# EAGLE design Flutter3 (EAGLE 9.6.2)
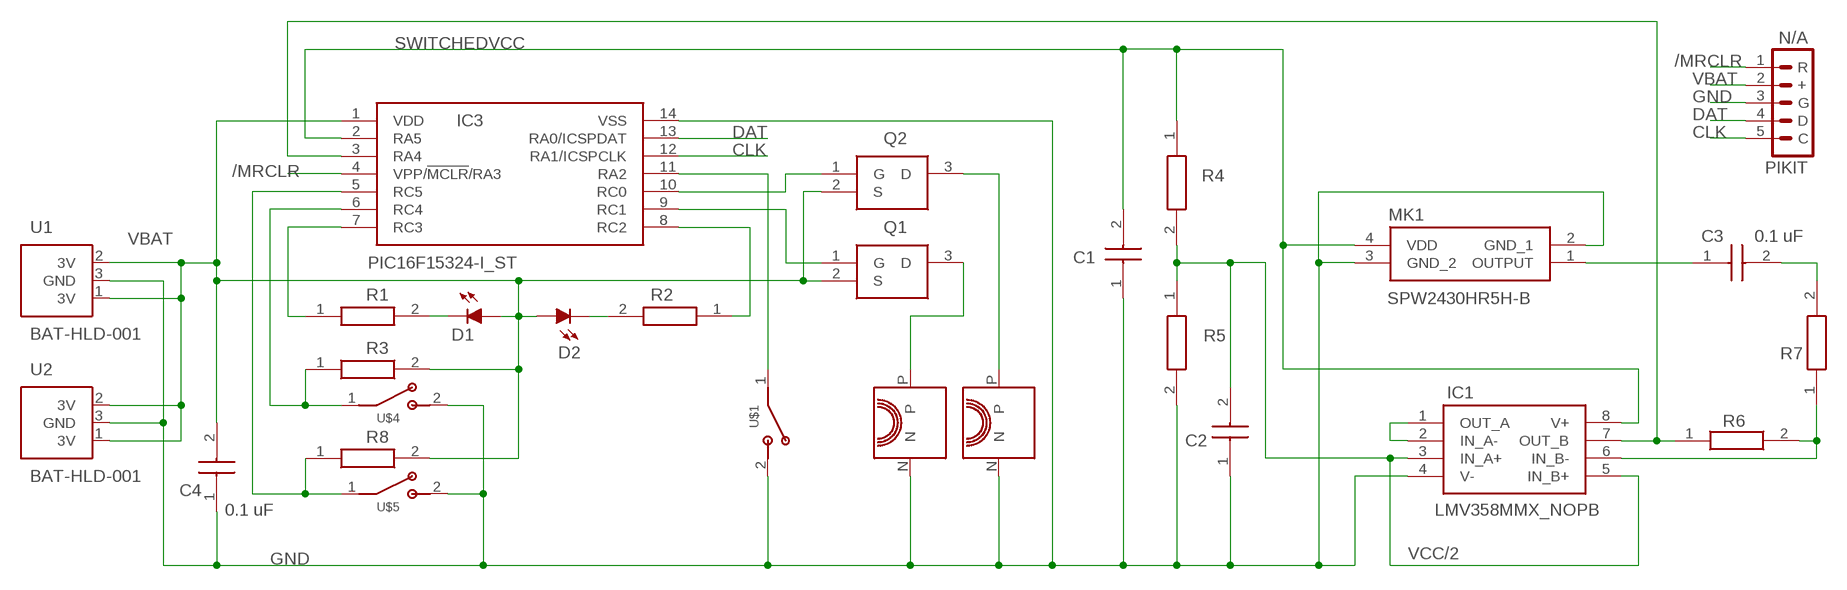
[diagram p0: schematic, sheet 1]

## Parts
C1  10 uF  C0805C106K8PACTU  [CAPC2013X140N]
C2  1.0 uF  CC0603KRX7R7BB104  [CAPC1608X90N]
C3  0.1 uF  CC0603KRX7R7BB104  [CAPC1608X90N]
C4  0.1 uF  CC0603KRX7R7BB104  [CAPC1608X90N]
D1  LEDCHIPLED_0805  [CHIPLED_0805]
D2  LEDCHIPLED_0805  [CHIPLED_0805]
IC1  LMV358MMX_NOPB  [SOP65P490X110-8N]
IC3  PIC16F15324-I_ST  [SOP65P640X120-14N]
MK1  SPW2430HR5H-B  [SPW2430HR5HB]
PIKIT  N/A  PICKIT  [MA05-1]
Q1  NTR4171PT1G  [SOT96P237X111-3N]
Q2  NTR4171PT1G  [SOT96P237X111-3N]
R1  220  CRCW0603240RFKEB  [RESC1608X50N]
R2  220  CRCW0603240RFKEB  [RESC1608X50N]
R3  220  CRCW0603240RFKEB  [RESC1608X50N]
R4  10 K  CRCW0603240RFKEB  [RESC1608X50N]
R5  10 K  CRCW0603240RFKEB  [RESC1608X50N]
R6  100 K  CRCW0603240RFKEB  [RESC1608X50N]
R7  1K  CRCW0603240RFKEB  [RESC1608X50N]
R8  220  CRCW0603240RFKEB  [RESC1608X50N]
U1  BAT-HLD-001  [BATHLD001]
U2  BAT-HLD-001  [BATHLD001]
U$1  SW-MOTION  [AF-1766]
U$2  VIBRATEFLAT  [PL-28821]
U$3  VIBRATEFLAT  [PL-28821]
U$4  SW-MOTIONFINGER  [FINGER-SW-12MM]
U$5  SW-MOTIONFINGER  [FINGER-SW-12MM]

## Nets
/MRCLR: IC3.4(VPP/!MCLR!/RA3) PIKIT.1(R)
CLK: IC3.12(RA1/ICSPCLK) PIKIT.5(C)
DAT: IC3.13(RA0/ICSPDAT) PIKIT.4(D)
GND: C1.1(C1) C2.1(C1) C4.1(C1) IC1.4(V-) IC3.14(VSS) MK1.2(GND_1) MK1.3(GND_2) PIKIT.3(G) R5.2 U1.3(GND) U2.3(GND) U$1.2 U$2.N U$3.N U$4.2 U$5.2
MIKIN: IC1.7(OUT_B) IC3.3(RA4) R6.1
N$1: IC1.1(OUT_A) IC1.2(IN_A-)
N$2: IC3.10(RC0) Q2.1(G)
N$3: IC3.9(RC1) Q1.1(G)
N$4: IC3.8(RC2) R2.1
N$5: IC3.5(RC5) R8.1 U$5.1
N$6: IC3.11(RA2) U$1.1
N$7: Q1.3(D) U$2.P
N$8: IC3.7(RC3) R1.1
N$9: Q2.3(D) U$3.P
N$10: D1.C R1.2
N$11: C3.1(C1) MK1.1(OUTPUT)
N$12: D2.C R2.2
N$13: C3.2(C2) R7.2
N$16: IC1.6(IN_B-) R6.2 R7.1
N$17: IC3.6(RC4) R3.1 U$4.1
SWITCHEDVCC: C1.2(C2) IC1.8(V+) IC3.2(RA5) MK1.4(VDD) R4.1
VBAT: C4.2(C2) D1.A D2.A IC3.1(VDD) PIKIT.2(+) Q1.2(S) Q2.2(S) R3.2 R8.2 U1.1(3V) U1.2(3V) U2.1(3V) U2.2(3V)
VCC/2: C2.2(C2) IC1.3(IN_A+) IC1.5(IN_B+) R4.2 R5.1

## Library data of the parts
C1 = SamacSys_Parts:C0805C106K8PACTU: CAPACITOR, 0805 10uF +/-10% 10V; ALLIED_NUMBER: 70096892; ALLIED_PRICE-STOCK: https://www.alliedelec.com/kemet-c0805c106k8pactu/70096892/; DESCRIPTION: CAPACITOR, 0805 10uF +/-10% 10V; HEIGHT: mm; MANUFACTURER_NAME: Kemet; MANUFACTURER_PART_NUMBER: C0805C106K8PACTU; MOUSER_PART_NUMBER: 80-C0805C106K8P; MOUSER_PRICE-STOCK: https://www.mouser.com/Search/Refine.aspx?Keyword=80-C0805C106K8P; RS_PART_NUMBER: 8692159; RS_PRICE-STOCK: https://uk.rs-online.com/web/p/products/8692159
C2-C4 = SamacSys_Parts:CC0603KRX7R7BB104: CAPACITOR, 0603 100nF +/-10% 16V; DESCRIPTION: CAPACITOR, 0603 100nF +/-10% 16V; HEIGHT: mm; MANUFACTURER_NAME: YAGEO (PHYCOMP); MANUFACTURER_PART_NUMBER: CC0603KRX7R7BB104; MOUSER_PART_NUMBER: 603-CC603KRX7R7BB104; MOUSER_PRICE-STOCK: https://www.mouser.com/Search/Refine.aspx?Keyword=603-CC603KRX7R7BB104; RS_PART_NUMBER: 6698763; RS_PRICE-STOCK: http://uk.rs-online.com/web/p/products/6698763
D1 D2 = philbot:LED: LED
IC1 = SamacSys_Parts:LMV358MMX_NOPB: General Purpose, Low Voltage, Rail-to-Rail Output Operational Amplifiers Source: Datasheet; DESCRIPTION: General Purpose, Low Voltage, Rail-to-Rail Output Operational Amplifiers; HEIGHT: 1.1mm; MANUFACTURER_NAME: Texas Instruments; MANUFACTURER_PART_NUMBER: LMV358MMX/NOPB; MOUSER_PART_NUMBER: 926-LMV358MMX/NOPB; MOUSER_PRICE-STOCK: https://www.mouser.com/Search/Refine.aspx?Keyword=926-LMV358MMX%2FNOPB
IC3 = SamacSys_Parts:PIC16F15324-I_ST: 8-bit Microcontrollers - MCU 7KB, 512B RAM, 4xPWMs, Comparator, DAC, ADC, 4xCLC, CWG, 2xEUSART, SPI/I2C Source: Datasheet; ARROW_PART_NUMBER: PIC16F15324-I/ST; ARROW_PRICE-STOCK: https://www.arrow.com/en/products/pic16f15324-ist/microchip-technology; DESCRIPTION: 8-bit Microcontrollers - MCU 7KB, 512B RAM, 4xPWMs, Comparator, DAC, ADC, 4xCLC, CWG, 2xEUSART, SPI/I2C; HEIGHT: 1.2mm; MANUFACTURER_NAME: Microchip; MANUFACTURER_PART_NUMBER: PIC16F15324-I/ST; MOUSER_PART_NUMBER: 579-PIC16F15324-I/ST; MOUSER_PRICE-STOCK: https://www.mouser.co.uk/ProductDetail/Microchip-Technology/PIC16F15324-I-ST?qs=IP4CA2YhK0DBTKI1lVIGkw%3D%3D
MK1 = SamacSys_Parts:SPW2430HR5H-B: MEMS Microphones MEMS Microphone Source: Datasheet; DESCRIPTION: MEMS Microphones MEMS Microphone; HEIGHT: 1mm; MANUFACTURER_NAME: Knowles; MANUFACTURER_PART_NUMBER: SPW2430HR5H-B; MOUSER_PART_NUMBER: 721-SPW2430HR5HB; MOUSER_PRICE-STOCK: https://www.mouser.com/Search/Refine.aspx?Keyword=721-SPW2430HR5HB
PIKIT = philbot:PICKIT: PIN HEADER; OC_FARNELL: unknown; OC_NEWARK: unknown
Q1 Q2 = BluJoy-e:NTR4171PT1G: Power MOSFET Source: Datasheet; ARROW_PART_NUMBER: NTR4171PT1G; ARROW_PRICE-STOCK: https://www.arrow.com/en/products/ntr4171pt1g/on-semiconductor; DESCRIPTION: Power MOSFET; HEIGHT: 1.11mm; MANUFACTURER_NAME: ON Semiconductor; MANUFACTURER_PART_NUMBER: NTR4171PT1G; MOUSER_PART_NUMBER: 863-NTR4171PT1G; MOUSER_PRICE-STOCK: https://www.mouser.co.uk/ProductDetail/ON-Semiconductor/NTR4171PT1G?qs=N5dOQkml4H8L27wHnYyw3w%3D%3D
R1-R8 = SamacSys_Parts:CRCW0603240RFKEB: Thick Film Resistors - SMD 1/10watt 240ohms 1%; DESCRIPTION: Thick Film Resistors - SMD 1/10watt 240ohms 1%; HEIGHT: 0.5mm; MANUFACTURER_NAME: Vishay; MANUFACTURER_PART_NUMBER: CRCW0603240RFKEB; MOUSER_PART_NUMBER: 71-CRCW0603240RFKEB; MOUSER_PRICE-STOCK: https://www.mouser.com/Search/Refine.aspx?Keyword=71-CRCW0603240RFKEB
U1 U2 = philbot:BAT-HLD-001: Coin Cell Battery Holders Linx CR2032 Battery Holder Source: Datasheet; DESCRIPTION: Coin Cell Battery Holders Linx CR2032 Battery Holder; HEIGHT: 4mm; MANUFACTURER_NAME: Linx Technologies; MANUFACTURER_PART_NUMBER: BAT-HLD-001; MOUSER_PART_NUMBER: 712-BAT-HLD-001; MOUSER_PRICE-STOCK: https://www.mouser.com/Search/Refine.aspx?Keyword=712-BAT-HLD-001
U$1 U$4 U$5 = philbot:SW-MOTION
U$2 U$3 = philbot:VIBRATE

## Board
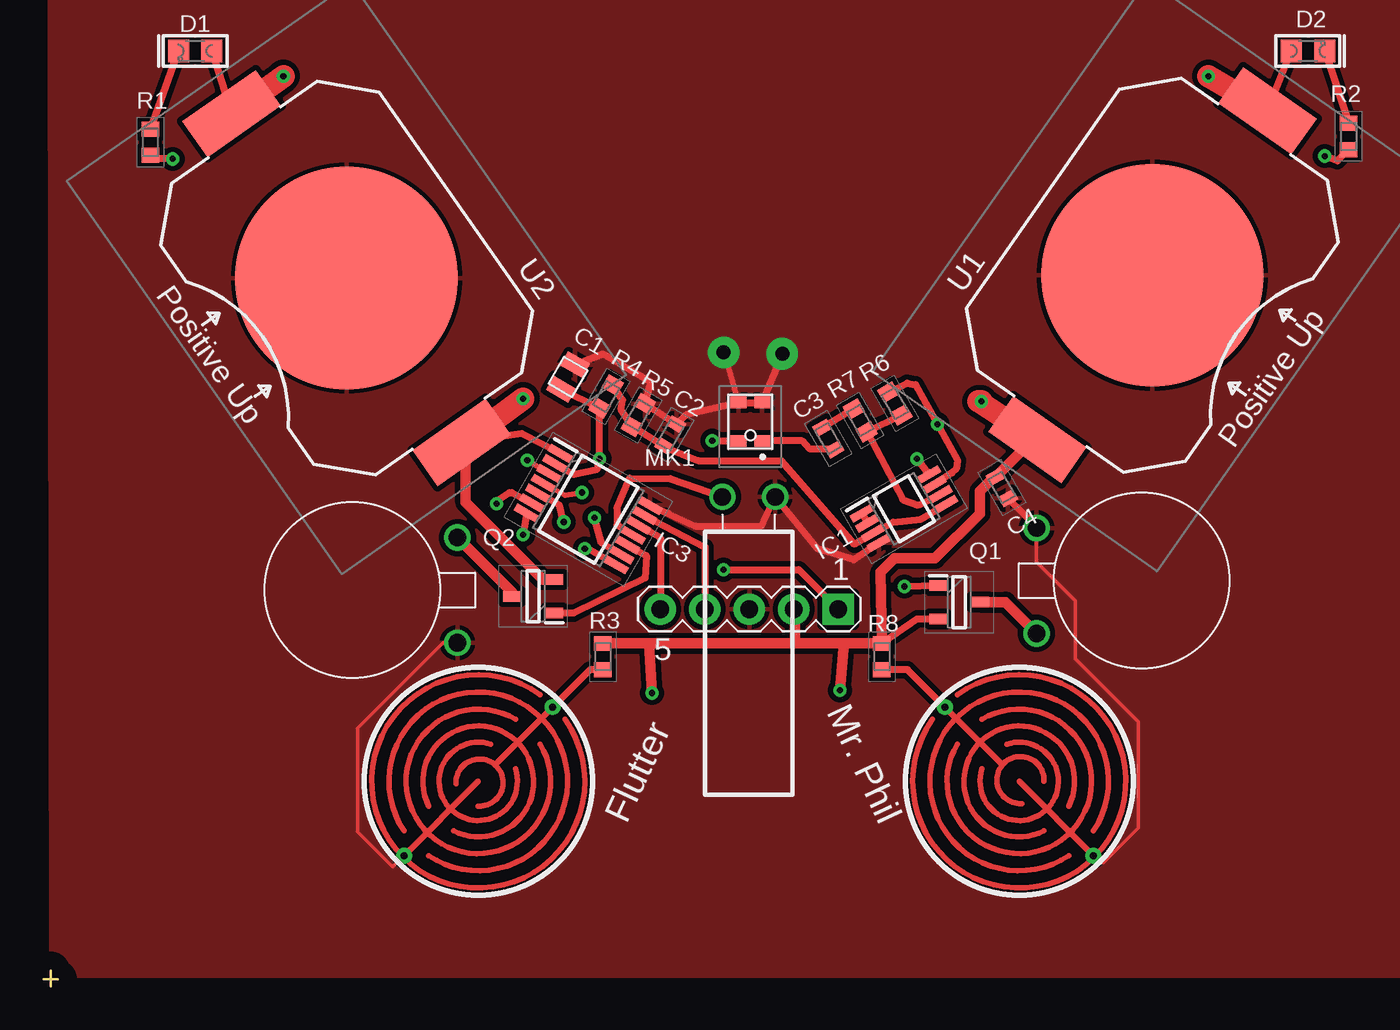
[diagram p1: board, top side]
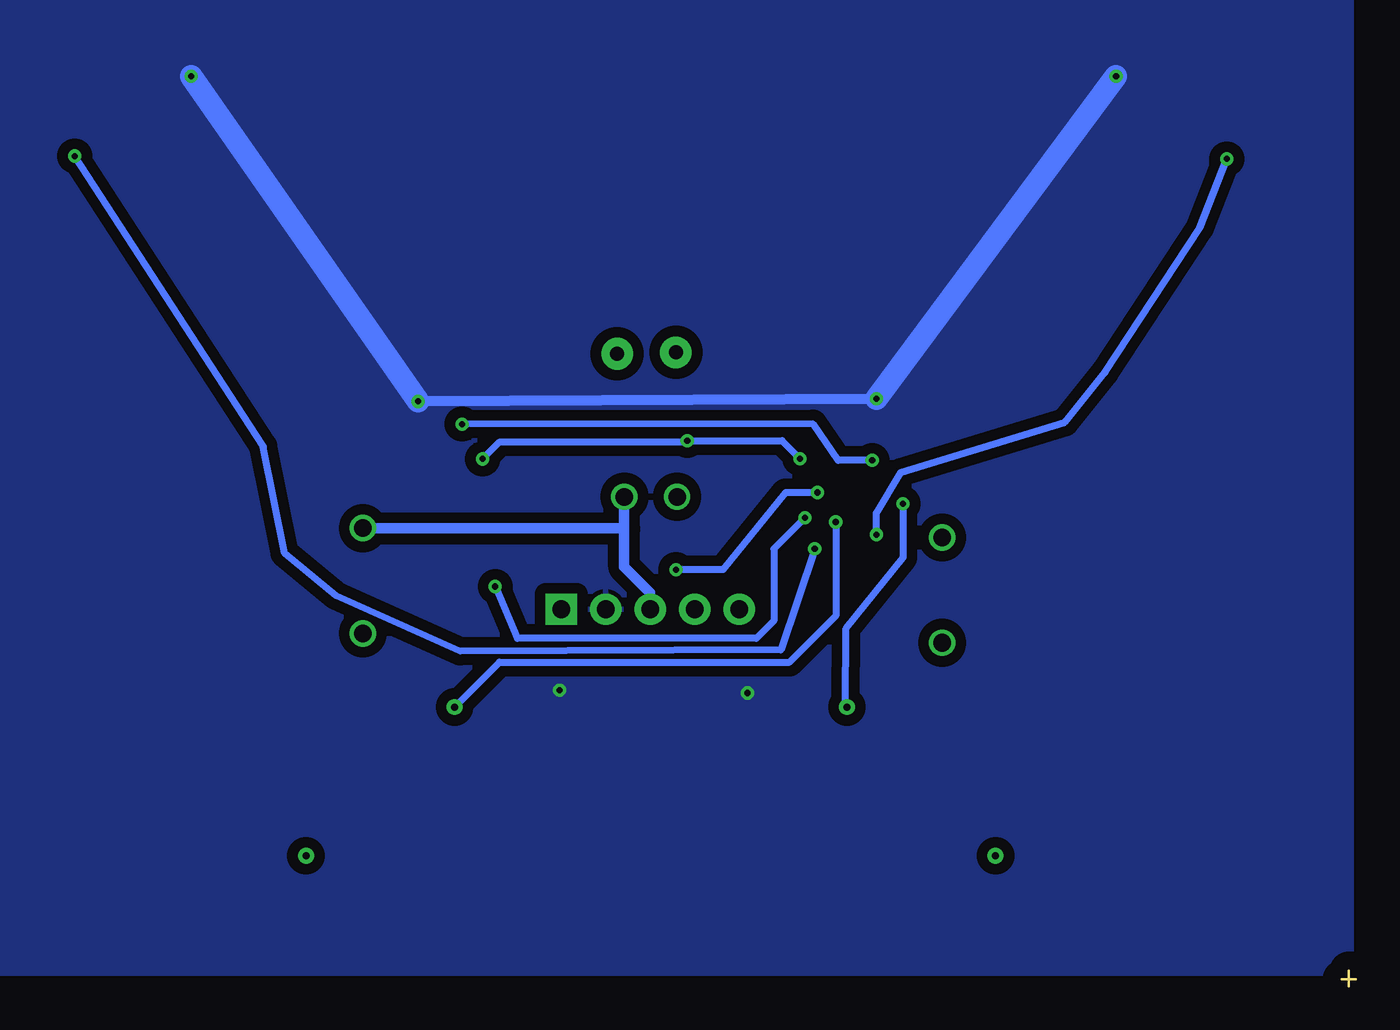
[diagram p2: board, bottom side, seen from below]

Size 0.8 x 0.88 mm. Coordinates in mm from the lower left corner, seen from the top.
Outline: 0,0.4 0.8,0.4
Outline: 0.4,0.88 0.4,0
Copper layers (1*16): Top 0.035mm / dielectric 1.5mm / Bottom 0.035mm
Design rules "default": minimum track width 6mil, minimum drill 0.35mm, track to track 6mil, track to pad 6mil, pad to pad 6mil, via to via 6mil, smd to smd 6mil, copper to edge 40mil, drill to drill 6mil, minimum pad ring 10mil, minimum via ring 8mil, stop-mask expansion 4mil, vias tented up to drill 0mil, thermal gap 10mil

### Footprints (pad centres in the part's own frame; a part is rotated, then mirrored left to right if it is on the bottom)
CAPC2013X140N = smd 0.914 x 1.448: 1 -0.813,0; 2 0.813,0
CAPC1608X90N = smd 0.66 x 0.94: 1 -0.711,0; 2 0.711,0
CHIPLED_0805 = smd 1.3 x 1.2: A 0,-0.953; C 0,0.953
SOP65P490X110-8N = smd 1.4 x 0.45: 1 -2.2,0.975; 2 -2.2,0.325; 3 -2.2,-0.325; 4 -2.2,-0.975; 5 2.2,-0.975; 6 2.2,-0.325; 7 2.2,0.325; 8 2.2,0.975
SOP65P640X120-14N = smd 1.475 x 0.45: 1 -2.938,1.95; 2 -2.938,1.3; 3 -2.938,0.65; 4 -2.938,0; 5 -2.938,-0.65; 6 -2.938,-1.3; 7 -2.938,-1.95; 8 2.938,-1.95; 9 2.938,-1.3; 10 2.938,-0.65; 11 2.938,0; 12 2.938,0.65; 13 2.938,1.3; 14 2.938,1.95
SPW2430HR5HB = smd 0.9 x 0.66: 1 -0.675,1.095; 2 -0.675,-1.095; 3 0.675,-1.095; 4 0.675,1.095
MA05-1 = drill 1.016 pad 1.778 square: 1 -5.08,0 | drill 1.016 pad 1.778: 2 -2.54,0; 3 0,0; 4 2.54,0; 5 5.08,0
SOT96P237X111-3N = smd 1 x 0.6: 1 -1.2,0.955; 2 -1.2,-0.955; 3 1.2,0
RESC1608X50N = smd 0.85 x 1: 1 -0.75,0; 2 0.75,0
BATHLD001 = smd 2.5 x 5.1: 1 11.45,0; 2 -11.45,0 | smd 12.7 x 12.7: 3 0,0
AF-1766 = drill 1: 1 9,1; 2 9,-2
PL-28821 = drill 1: N 6,-3; P 6,3
FINGER-SW-12MM = drill 0.4: 1 0,6; 2 0,-6

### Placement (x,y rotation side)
C1  29.92,34.76 240 top  (outside the outline)
C2  35.76,31.43 240 top  (outside the outline)
C3  44.78,31.24 120 top  (outside the outline)
C4  54.69,28.45 120 top  (outside the outline)
D1  8.64,53.36 90 top  (outside the outline)
D2  72.16,53.36 270 top  (outside the outline)
IC1  49.1,27.24 30 top  (outside the outline)
IC3  31.08,27.21 330 top  (outside the outline)
MK1  40.33,32.2 180 top  (outside the outline)
PIKIT  40.27,21.51 180 top  (outside the outline)
Q1  52.25,21.91 0 top  (outside the outline)
Q2  27.93,22.24 180 top  (outside the outline)
R1  6.09,48.15 90 top  (outside the outline)
R2  74.48,48.48 90 top  (outside the outline)
R3  31.92,18.8 90 top  (outside the outline)
R4  32.1,33.65 60 top  (outside the outline)
R5  33.94,32.58 60 top  (outside the outline)
R6  48.58,33.24 300 top  (outside the outline)
R7  46.6,32.28 120 top  (outside the outline)
R8  47.84,18.8 90 top  (outside the outline)
U1  63.28,40.56 55 top  (outside the outline)
U2  17.28,40.4 305 top  (outside the outline)
U$1  39.74,18.92 90 top  (outside the outline)
U$2  62.67,23.13 180 top  (outside the outline)
U$3  17.61,22.59 0 top  (outside the outline)
U$4  24.8,11.68 315 top  (outside the outline)
U$5  55.68,11.68 45 top  (outside the outline)

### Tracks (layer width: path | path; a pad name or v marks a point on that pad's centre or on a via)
/MRCLR  (via drill 0.35)
  Top 0.305: IC3.4 29.76,28 v30.72,28.16
  Top 0.406: v38.8,23.76 43.1,23.76 PIKIT.1
  Bottom 0.406: v30.72,28.16 32.55,28.16 36.12,23.76 v38.8,23.76
CLK
  Top 0.406: IC3.12 35.2,25.6 PIKIT.5
DAT
  Top 0.406: IC3.13 37.76,25.04 PIKIT.4
GND  (via drill 0.8 pad 1.8)
  Top 0.2: U$4.2 19.92,6.8 17.92,8.8 17.92,14.72 22.79,19.59 U$3.N | U$5.2 60.08,7.44 60.48,7.04 62.48,9.04 62.48,15.08 58.88,18.68 58.88,22 56.67,24.21 U$2.N
  Top 0.305: MK1.3 38.85,36.11 v38.8,36.16
  Top 0.406: U$2.N 56.39,26.49 C4.1 | 35.68,26.96 IC3.14 37.2,26.24 40.97,26.24 U$1.2 44.16,24.96 46.24,24.32 IC1.4 | v42.16,36.08 MK1.2 MK1.3 36.66,32.59 C2.1 R5.2 34.64,34.48 31.92,36.08 C1.1
  Bottom 0.61: PIKIT.3 40.27,22.43 41.76,23.92 41.76,26.08 | 41.76,26.08 41.76,27.9 U$1.2 | U$2.N 41.81,26.13 41.76,26.08
  pour Top (isolate 0.3): 0.32,57.12 80.56,57.12 80.56,0.56 0.4,0.56
MIKIN  (via drill 0.35)
  Top 0.305: IC3.3 v27.6,30
  Top 0.406: R6.1 49.28,34.4 49.76,34.32 v51.01,32.06 52.16,30 52.08,29.52 51.84,29.28 IC1.7
  Bottom 0.406: v27.6,30 29.55,30 30.99,32.08 v51.01,32.06
N$1
  Top 0.406: IC1.1 IC1.2
N$2
  Top 0.406: IC3.10 34.4,24.56 34.32,23.28 30.24,21.28 Q2.1
N$3  (via drill 0.35)
  Top 0.406: IC3.9 31.84,25.28 v31.44,26.72 | v49.12,22.8 Q1.1
  Bottom 0.406: v31.44,26.72 33.21,24.95 33.21,20.84 34.21,19.84 47.85,19.84 49.07,22.75 v49.12,22.8
N$4  (via drill 0.35)
  Top 0.406: IC3.8 30.94,25 v30.88,24.96 | R2.1 73.84,47.09 v73.12,47.36
  Bottom 0.406: v30.88,24.96 32.81,19.18 51.12,19.11 58.2,22.28 61.13,24.68 62.35,30.79 62.37,30.79 v73.12,47.36
N$5  (via drill 0.35)
  Top 0.406: U$5.1 49.31,18.05 R8.1 | v29.68,26.48 29.44,27.44 IC3.5
  Bottom 0.406: U$5.1 48.88,18.48 32.32,18.48 29.68,21.12 v29.68,26.48
N$6
  Top 0.406: IC3.11 32.72,26.32 32.72,27.28 33.44,28.99 35.76,28.96 U$1.1
N$7
  Top 0.61: Q1.3 54.89,21.91 U$2.P
N$8  (via drill 0.35)
  Top 0.406: IC3.7 v27.36,25.76 | v7.36,47.2 6.29,47.2 R1.1
  Bottom 0.406: v27.36,25.76 27.36,26.99 25.97,29.31 16.61,32.18 14.31,35.02 8.9,43.28 v7.36,47.2
N$9
  Top 0.61: U$3.P 26.73,22.47 Q2.3
N$10
  Top 0.406: R1.2 D1.C
N$11
  Top 0.406: C3.1 45.12,30.64 43.75,30.64 43.31,31.1 MK1.1
N$12
  Top 0.406: D2.C R2.2
N$13
  Top 0.406: C3.2 R7.2
N$16
  Top 0.406: R6.2 R7.1 49.04,27.76 49.92,27.44 IC1.6
N$17  (via drill 0.35)
  Top 0.406: R3.1 31.21,18.05 31.14,18.02 U$4.1 | v25.84,27.52 25.78,27.65 26.56,28.16 26.72,28.16 IC3.6
  Bottom 0.406: U$4.1 29.13,16.01 29.09,20.41 25.84,24.45 v25.84,27.52
SWITCHEDVCC  (via drill 0.35)
  Top 0.406: C1.2 R4.1 v31.73,30.1 31.6,29.5 30.24,29.2 IC3.2 | v38.16,31.12 MK1.4 | v49.84,30.08 IC1.8
  Bottom 0.406: v31.73,30.1 32.75,31.12 v38.16,31.12 38.23,31.05 48.87,31.05 v49.84,30.08
VBAT  (via drill 0.35)
  Top 0.406: D1.A U2.2 | D2.A U1.1 | IC3.1 27.28,31.52 24.32,31.09 24.05,31.05 U2.1 | Q1.2 49.86,20.95 R8.2
  Top 0.61: R3.2 34.56,19.55 | 34.56,19.55 42.88,19.55 | 42.88,19.55 45.68,19.55 | 45.68,19.55 R8.2 47.76,23.6 48.56,24.4 50.88,24.4 53.44,26.96 53.44,28.24 54.27,29.07 C4.2 56.45,31.18 U1.2 | PIKIT.2 42.88,21.44 42.88,19.55 | Q2.2 28.48,23.2 24.08,27.6 24.08,30.85 24.32,31.09 | 34.56,19.55 v34.72,16.72 | 45.68,19.55 v45.44,16.88
  Top 1.27: U2.2 v13.68,51.92 | v27.36,33.52 24.05,31.05 | U1.2 53.36,33.36 v53.52,33.36 | v66.48,51.92 U1.1
  Bottom 0.61: v27.36,33.52 v53.52,33.36
  Bottom 1.27: v13.68,51.92 v27.36,33.52 | v53.52,33.36 v66.48,51.92
  pour Bottom (isolate 0.61): 0.24,57.2 0.24,0.72 80.4,0.72 80.4,57.2
VCC/2
  Top 0.406: IC1.5 50.08,26.64 48.48,26.48 IC1.3 46.27,25.22 42.1,29.99 37.34,29.99 35.51,30.71 C2.2 R5.1 32.96,32.88 33.04,33.44 R4.2

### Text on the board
tNames: Flutter | Mr. Phil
